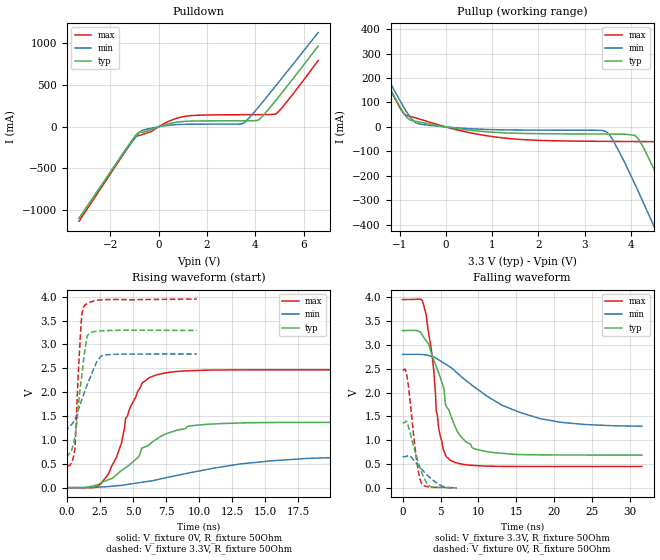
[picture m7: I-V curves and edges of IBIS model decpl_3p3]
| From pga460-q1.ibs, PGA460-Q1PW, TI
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|   decpl_3p3 Model
[Model]   decpl_3p3
Model_type   Output
Polarity   Non-Inverting
Vmeas = 1.65
Vref = 0
Cref = 2pF
Rref = 150
|   typ   min   max
|   (nom PVT)   (fast PVT)   (slow PVT)
C_comp   1.625e-12   1.625e-12   1.667e-12
| Where nom  PVT is Nominal Process, 3.3V, 27C
|   Fast PVT is Strong Process,  3.95V, -40C
|   Slow PVT is Weak Process,   2.8V, 125C
[Voltage Range]   3.3   2.8   3.95
|Junction Temperature
[Temperature Range]   27   125   -40
[Pullup Reference]   3.3   2.8   3.95
[Pulldown Reference]   0   0   0
[Power Clamp Reference]   3.3   2.8   3.95
[GND Clamp Reference]   0   0   0
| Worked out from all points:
|   slope of the pulldown table from 0 to 0.495 V, typ, clamps not added: 11.9 ohm
|   slope of the pullup table from 0 to 0.495 V, typ, clamps not added: 38.7 ohm
|   falling waveform, V_fixture 3.3V, R_fixture 50Ohm: 20-80 % time 3.24ns typ, 8.72ns min, 1.47ns max; typ from 3.3 V to 0.689 V
|   rising waveform, V_fixture 0V, R_fixture 50Ohm: 20-80 % time 3.48ns typ, 8ns min, 1.83ns max; typ from 0 V to 1.37 V
|   rising waveform, V_fixture 3.3V, R_fixture 50Ohm: 20-80 % time 624ps typ, 1.22ns min, 362ps max; typ from 0.689 V to 3.29 V
|   falling waveform, V_fixture 0V, R_fixture 50Ohm: 20-80 % time 1.55ns typ, 2.44ns min, 1.05ns max; typ from 1.37 V to 0.002 V
[Pulldown]
|   Voltage   I(typ)   I(min)   I(max)
-3.3V     -1.1A      -1.096A    -1.133A
-1.158V   -181.2mA   -198.7mA   -198.9mA
-890.5mV  -81.85mA   -98mA      -108.1mA
-630.3mV  -63.82mA   -37.09mA   -88.04mA
-329.6mV  -35.03mA   -18.82mA   -59.31mA
460.4mV   39.65mA    19.51mA    71.88mA
1.061V    64.49mA    29.45mA    124.1mA
3.498V    72.71mA    43.1mA     145mA
4.155V    87.91mA    245.9mA    145.7mA
4.896V    335.1mA    510.4mA    164.3mA
5.505V    558.1mA    730.5mA    374.1mA
6.6V      968.4mA    1.13A      794.4mA
[Pullup]
|   Voltage   I(typ)   I(min)   I(max)
-3.3V     940.5mA    941.1mA    969.1mA
-1.551V   281.5mA    302.1mA    285.7mA
-948mV    66.04mA    91.44mA    63.16mA
-572.8mV  19.57mA    11.63mA    32.19mA
1.251V    -24.15mA   -11.92mA   -45.29mA
3.47V     -29.08mA   -20.06mA   -59.08mA
4.168V    -48.96mA   -265.6mA   -59.87mA
4.514V    -176.8mA   -410.4mA   -60.36mA
4.813V    -302mA     -536.7mA   -66.58mA
5.058V    -407.1mA   -640.3mA   -139.9mA
5.358V    -537.2mA   -767.3mA   -266.1mA
6.6V      -1.075A    -1.291A    -817mA
[Ramp]
R_load = 50
|   typ   min   max
dV/dt_r   0.82009/3.77118e-09   0.393391/7.10179e-09   1.48126/1.95963e-09
dV/dt_f   1.5668/3.50145e-09   0.910535/7.76753e-09   2.10035/1.5968e-09
[Falling Waveform]
V_fixture = 3.3V
V_fixture_min = 2.8V
V_fixture_max = 3.95V
R_fixture = 50Ohm
|   Time   V(typ)   V(min)   V(max)
0s        3.3V       2.8V       3.95V
2.624ns   3.202V     2.796V     3.924V
3.742ns   2.857V     2.764V     2.955V
4.424ns   2.551V     2.718V     1.626V
4.822ns   2.381V     2.68V      1.197V
6.229ns   1.575V     2.539V     584.6mV
7.917ns   1.038V     2.308V     495.7mV
10.92ns   766.1mV    1.947V     458.4mV
18.18ns   693.5mV    1.452V     449.5mV
31.52ns   688.7mV    1.293V     449.4mV
[Rising Waveform]
V_fixture = 0V
V_fixture_min = 0V
V_fixture_max = 0V
R_fixture = 50Ohm
|   Time   V(typ)   V(min)   V(max)
0s        176.3pV    1.319nV    283.8pV
2.624ns   104.3mV    13.18mV    98.73mV
3.742ns   269.6mV    37.36mV    635mV
4.116ns   355.1mV    46.78mV    928.4mV
4.424ns   416.8mV    59.85mV    1.44V
5.626ns   796.2mV    109.9mV    2.165V
6.926ns   1.041V     172.2mV    2.373V
9.562ns   1.301V     325mV      2.452V
18.18ns   1.366V     611.4mV    2.469V
39.52ns   1.367V     655.6mV    2.469V
[Rising Waveform]
V_fixture = 3.3V
V_fixture_min = 2.8V
V_fixture_max = 3.95V
R_fixture = 50Ohm
|   Time   V(typ)   V(min)   V(max)
0s        688.6mV    1.282V     449.4mV
321.7ps   774.4mV    1.319V     511.3mV
598.3ps   1.08V      1.433V     822.8mV
864.7ps   1.754V     1.634V     2.479V
1.049ns   2.202V     1.786V     3.38V
1.134ns   2.389V     1.855V     3.655V
1.336ns   2.856V     2.013V     3.82V
1.529ns   3.19V      2.155V     3.852V
2.578ns   3.284V     2.758V     3.934V
9.821ns   3.294V     2.8V       3.949V
[Falling Waveform]
V_fixture = 0V
V_fixture_min = 0V
V_fixture_max = 0V
R_fixture = 50Ohm
|   Time   V(typ)   V(min)   V(max)
0s        1.367V     655.7mV    2.469V
350.3ps   1.388V     656.4mV    2.486V
604.2ps   1.37V      668.9mV    2.315V
872.2ps   1.225V     675.9mV    1.994V
1.879ns   635.6mV    507.1mV    552.5mV
2.19ns    474.8mV    449.1mV    261.9mV
2.53ns    320.4mV    387.9mV    87.02mV
3.656ns   31.3mV     207.6mV    18.97mV
5.322ns   6.081mV    33.7mV     15.36mV
7.116ns   1.607mV    4.131mV    2.464mV
